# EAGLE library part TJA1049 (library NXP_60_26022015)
High-speed CAN transceiver with Standby mode The TJA1049 high-speed CAN transceiver provides an interface between a Controller Area Network (CAN) protocol controller and the physical two-wire CAN bus. The transceiver is designed for high-speed (up to 1 Mbit/s) CAN applications in the automotive industry, supplying the differential transmit and receive capability to (a microcontroller with) a CAN protocol controller. The TJA1049 belongs to the third generation of high-speed CAN transceivers from NXP Semiconductors, offering significant improvements over first- and second-generation devices such as the TJA1040. It offers improved ElectroMagnetic Compatibility (EMC) and ElectroStatic Discharge (ESD) performance, and also features: Ideal passive behavior to the CAN bus when the supply voltage is off A very low-current Standby mode with bus wake-up capability These features make the TJA1049 an excellent choice for all types of HS-CAN networks, in nodes that require a low-power mode with wake-up capability via the CAN bus. AAL Eindhoven MK
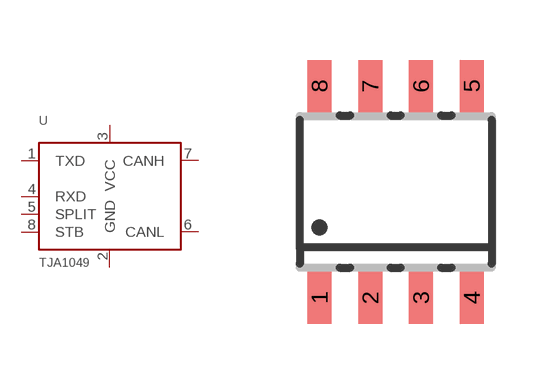
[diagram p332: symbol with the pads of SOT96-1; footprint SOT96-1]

Designator prefix U

## TJA1049T  [SOT96-1]
1  TXD  out
2  GND
3  VCC
4  RXD
5  SPLIT  pwr
6  CANL
7  CANH
8  STB  pas

## Footprint SOT96-1 (pad centres in mm)
SOT96-1 SO8: plastic small outline package; 8 leads; body width 3.9 mm JEDEC: MS-012 IEC: 076E03
smd 0.6 x 1.3: 1 -1.905,-2.65; 2 -0.635,-2.65; 3 0.635,-2.65; 4 1.905,-2.65; 5 1.905,2.65; 6 0.635,2.65; 7 -0.635,2.65; 8 -1.905,2.65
